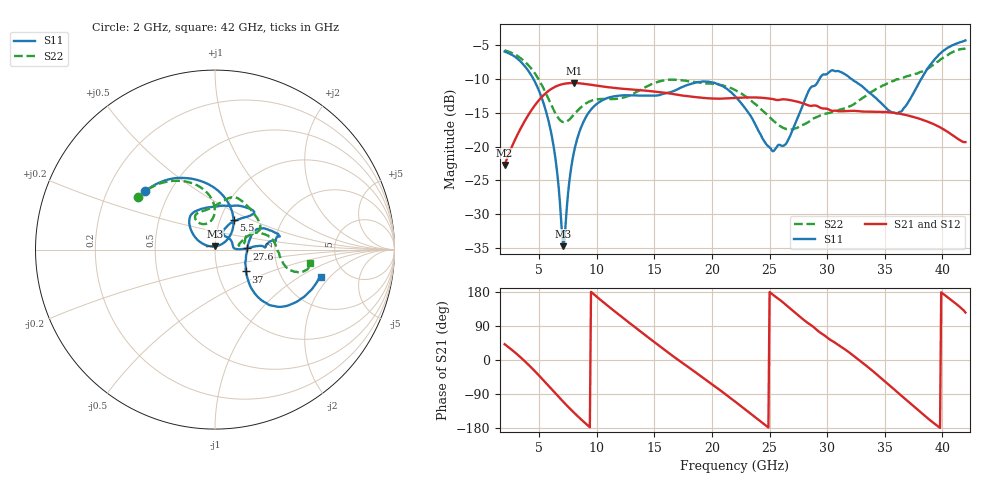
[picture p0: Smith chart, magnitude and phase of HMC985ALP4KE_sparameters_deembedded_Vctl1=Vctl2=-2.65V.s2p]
!s2p File: Measurements: S11, S21, S12, S22
# GHz S dB R 50.0
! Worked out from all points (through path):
!   401 points, 2 GHz to 42 GHz, reference 50 ohm
!   highest |S21| = -10.57 dB at 8 GHz (marker M1); lowest = -22.7 dB at 2 GHz (marker M2)
!   lowest |S11| = -34.7 dB at 7.1 GHz (marker M3), VSWR 1.04, Z = 49.9 + j1.82 ohm
!   |S11| at or under -10 dB: 4.513 GHz to 29.32 GHz (24.81 GHz wide, 147 % of centre); 32.14 GHz to 38.16 GHz (6.019 GHz wide, 17.1 % of centre)
!   |S22| runs from -17.5 to -5.4 dB; largest |S21 - S12| = 0.0003
!   S11 on the Smith chart (normalised r, x): 2 GHz: 0.37, +0.32; 5.5 GHz: 1.16, +0.40; 27.6 GHz: 1.43, +0.02; 37 GHz: 1.37, -0.35; 42 GHz: 3.30, -1.62
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2  -5.90 139.9  -22.72 41.7  -22.73 41.7  -5.72 145.8
3.7  -7.97 104.1  -16.34 -1.8  -16.35 -1.8  -7.33 117.0
5.5  -14.23 57.9  -12.18 -57.8  -12.19 -57.8  -11.80 91.7
6.3  -20.46 40.0  -11.20 -84.5  -11.21 -84.5  -14.70 92.4
7.1  -34.75 93.0  -10.71 -110.6  -10.71 -110.6  -16.36 106.5
8  -20.96 153.3  -10.57 -138.3  -10.57 -138.3  -15.30 120.6
8.7  -16.88 146.0  -10.65 -158.4  -10.65 -158.4  -14.06 122.8
10.1  -13.53 133.0  -10.98 164.4  -10.99 164.4  -12.97 116.8
12.2  -12.41 119.6  -11.41 113.0  -11.42 113.0  -12.78 98.3
15.4  -12.37 87.3  -11.92 37.9  -11.92 37.9  -10.35 73.1
18.2  -10.69 53.4  -12.58 -24.3  -12.59 -24.3  -10.35 55.1
22  -12.50 48.4  -12.77 -109.6  -12.78 -109.6  -11.60 23.0
25.3  -20.70 54.3  -12.95 172.2  -12.95 172.2  -16.12 17.6
26.5  -19.39 3.5  -13.03 143.1  -13.03 143.1  -17.41 11.4
27.6  -15.07 2.2  -13.42 115.0  -13.42 115.0  -17.01 9.0
28.7  -11.07 2.4  -13.94 89.8  -13.94 89.8  -15.95 11.1
31.1  -8.88 14.2  -14.76 37.0  -14.77 37.1  -14.53 23.1
33.3  -11.45 25.6  -14.81 -12.8  -14.82 -12.8  -12.54 23.3
35.4  -14.68 6.3  -14.90 -66.6  -14.91 -66.6  -10.52 15.8
37  -13.52 -35.2  -15.38 -108.8  -15.39 -108.8  -9.54 7.1
39.7  -6.38 -41.6  -17.04 -176.9  -17.03 -176.9  -7.29 -15.4
42  -4.26 -14.5  -19.32 125.2  -19.32 125.2  -5.45 -8.3
